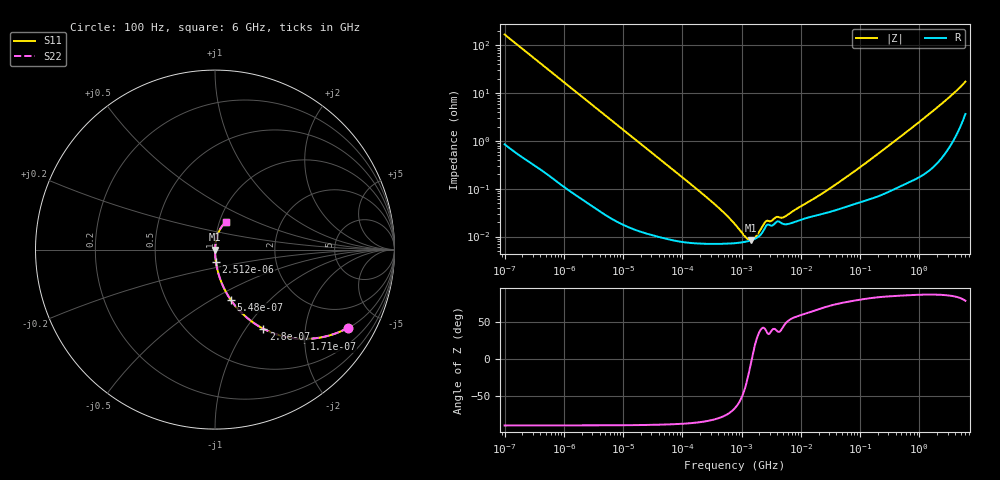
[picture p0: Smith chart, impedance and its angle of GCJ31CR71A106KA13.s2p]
!Murata Part Number: GCJ31CR71A106KA13
!These Parameters are Measured in Series Mode Connection
!Data Generated on Mar 13, 2026
!  o--ll--o
!Port1  Port2
!  o------o
!Operation Temp=25[degC], DC Bias Voltage=0[V]
!Freq. Start=100[Hz] Stop=6[GHz] 401[Steps]
# Hz S RI R 50
!Freq.(Hz) S11(Real) S11(Imag) S21(Real) S21(Imag) S12(Real) S12(Imag) S22(Real) S22(Imag)
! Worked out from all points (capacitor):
!   401 points, 100 Hz to 6 GHz, reference 50 ohm
!   read as one part in series: C = 9.39 uF near 109 Hz
!   lowest |Z| = 8.36 mohm at 1.45 MHz (marker M1)
!   series resonance near 1.49 MHz, so ESL is about 1.2 nH
!   S11 on the Smith chart (normalised r, x): 100 Hz: 1.02, -3.38; 171 Hz: 1.01, -1.98; 280 Hz: 1.01, -1.21; 548 Hz: 1.00, -0.62; 2.512 kHz: 1.00, -0.14; 6 GHz: 1.07, +0.34
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100  0.7402 -0.436  0.2598 0.436  0.2598 0.436  0.7402 -0.436
171  0.4953 -0.4974  0.5047 0.4974  0.5047 0.4974  0.4953 -0.4974
280  0.27 -0.4411  0.73 0.4411  0.73 0.4411  0.27 -0.4411
548  0.0894 -0.2823  0.9106 0.2823  0.9106 0.2823  0.0894 -0.2823
1026  0.0279 -0.1615  0.9721 0.1615  0.9721 0.1615  0.0279 -0.1615
2008  0.0078 -0.0845  0.9922 0.0845  0.9922 0.0845  0.0078 -0.0845
2512  0.00512 -0.0678  0.9949 0.0678  0.9949 0.0678  0.00512 -0.0678
7358  0.00076 -0.0234  0.9992 0.0234  0.9992 0.0234  0.00076 -0.0234
40335  0.000116 -0.00429  0.9999 0.00429  0.9999 0.00429  0.000116 -0.00429
316350  7.03e-05 -0.000527  0.9999 0.000527  0.9999 0.000527  7.03e-05 -0.000527
774597  7.25e-05 -0.000166  0.9999 0.000166  0.9999 0.000166  7.25e-05 -0.000166
1108252  7.67e-05 -7.14e-05  0.9999 7.14e-05  0.9999 7.14e-05  7.67e-05 -7.14e-05
1449809  8.33e-05 -6.6e-06  0.9999 6.6e-06  0.9999 6.6e-06  8.33e-05 -6.6e-06
1813585  9.44e-05 4.9e-05  0.9999 -4.9e-05  0.9999 -4.9e-05  9.44e-05 4.9e-05
2594782  0.000167 0.000129  0.9998 -0.000129  0.9998 -0.000129  0.000167 0.000129
3882480  0.000202 0.000159  0.9998 -0.000159  0.9998 -0.000159  0.000202 0.000159
5311619  0.000181 0.000185  0.9998 -0.000185  0.9998 -0.000185  0.000181 0.000185
1.555665e7  0.000263 0.000528  0.9997 -0.000528  0.9997 -0.000528  0.000263 0.000528
6.233367e7  0.000434 0.0018  0.9996 -0.0018  0.9996 -0.0018  0.000434 0.0018
3.124326e8  0.000939 0.0081  0.9991 -0.0081  0.9991 -0.0081  0.000939 0.0081
1.95892e9  0.00566 0.0485  0.9943 -0.0485  0.9943 -0.0485  0.00566 0.0485
6e9  0.0607 0.1542  0.9393 -0.1542  0.9393 -0.1542  0.0607 0.1542
